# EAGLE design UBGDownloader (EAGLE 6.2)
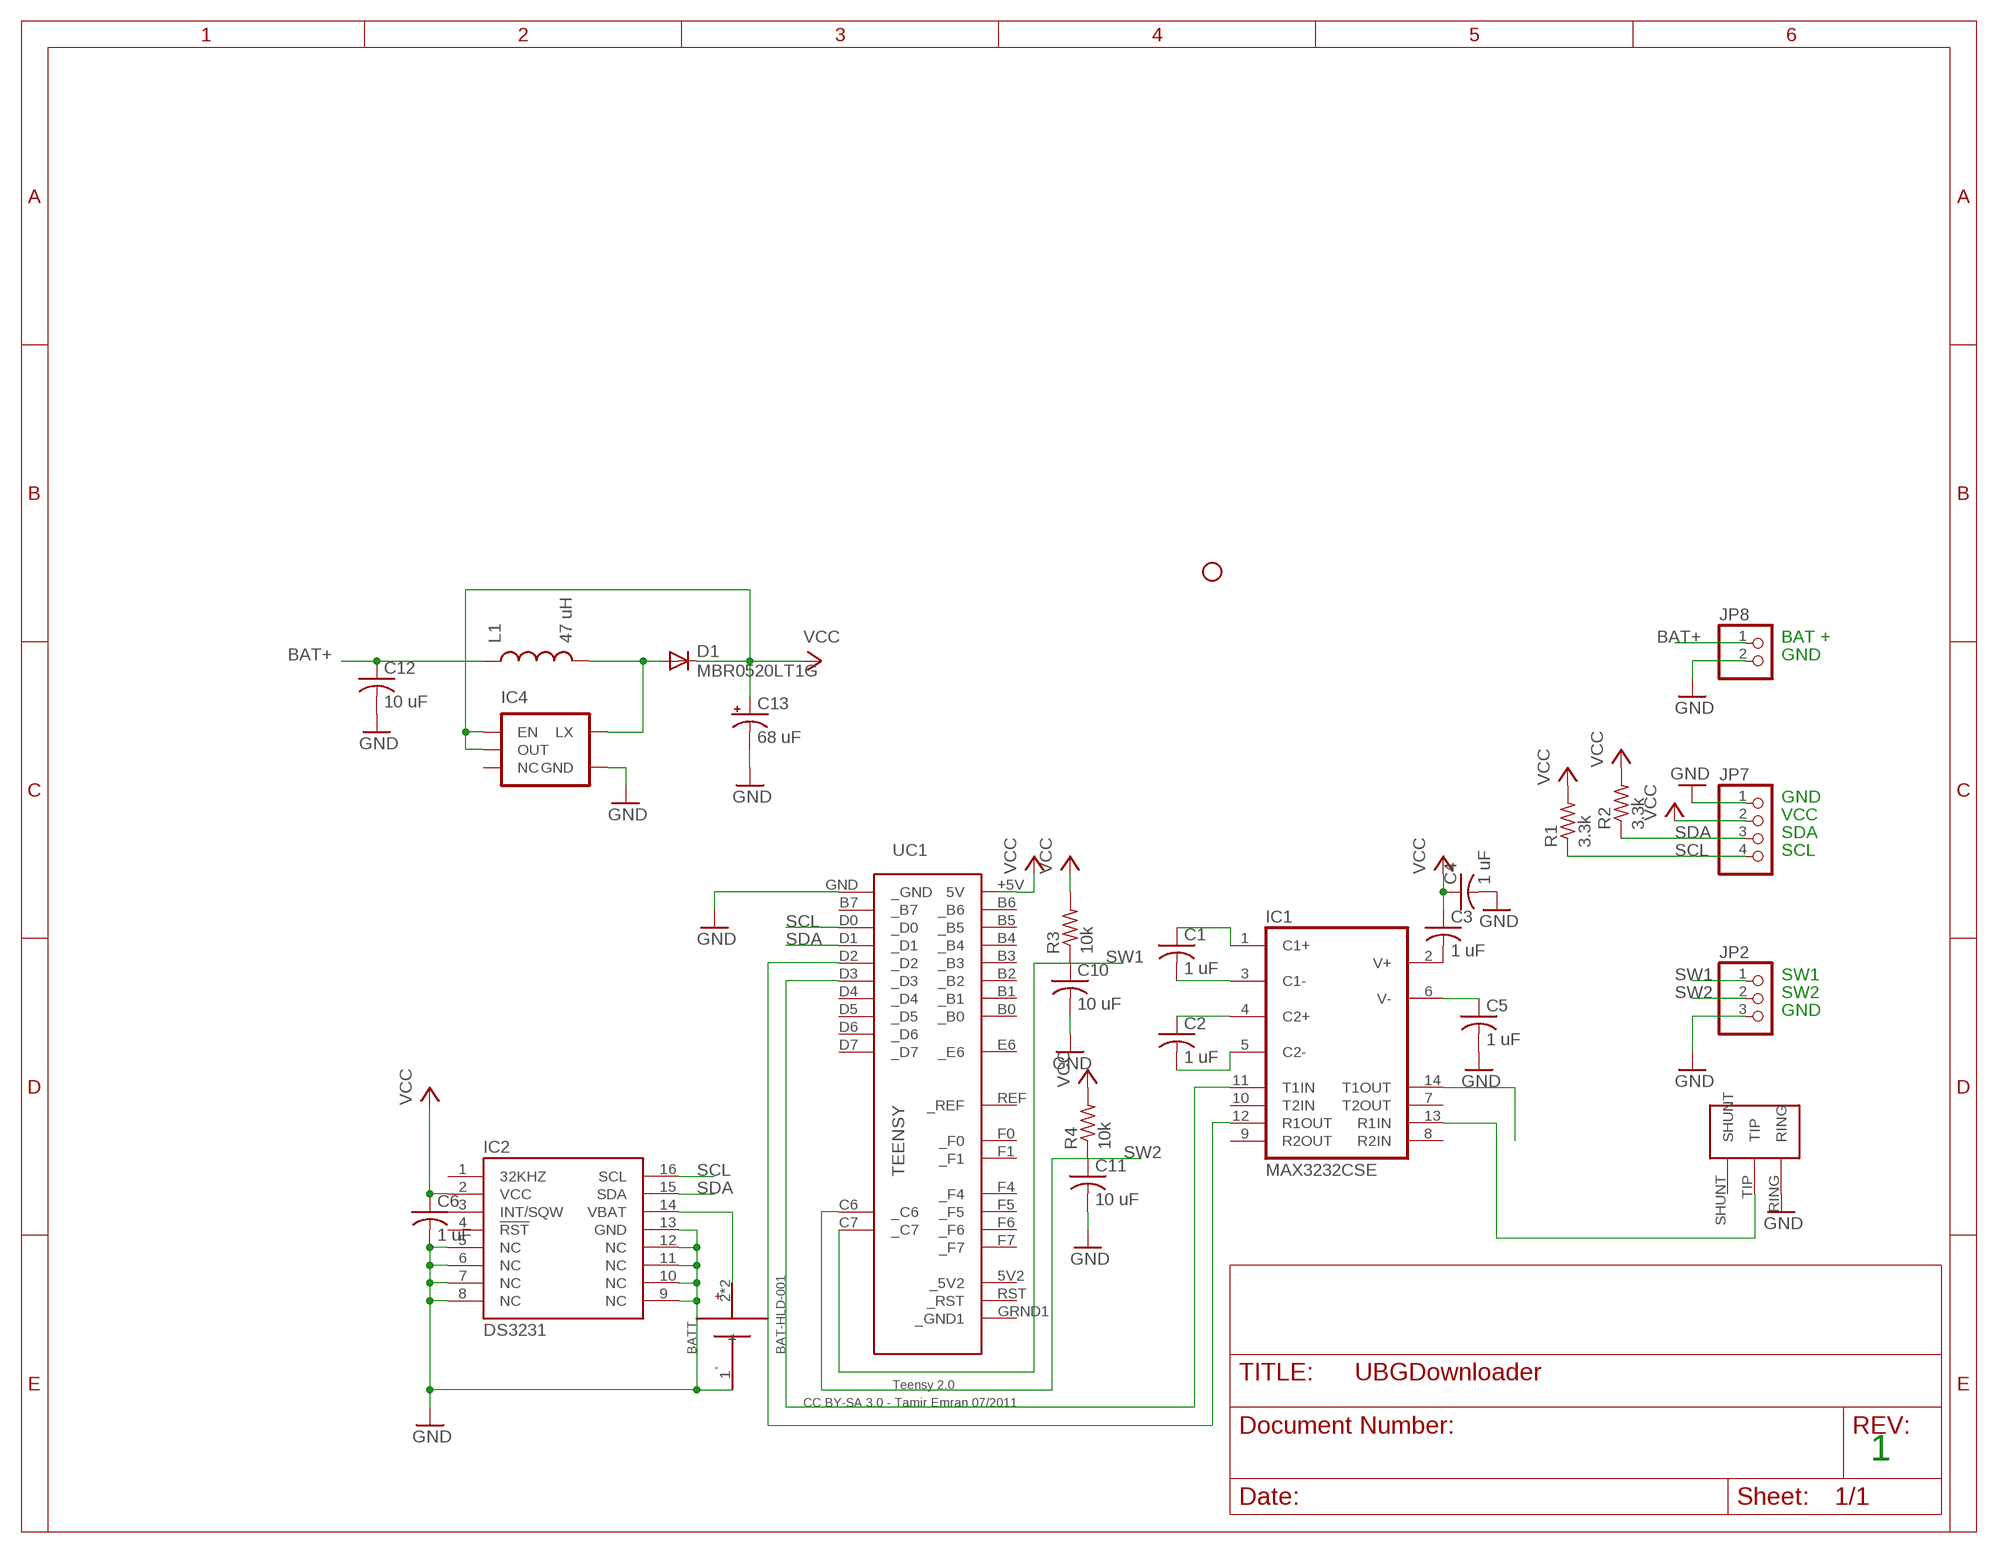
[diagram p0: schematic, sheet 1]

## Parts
BATT  BAT-HLD-001  [BAT-HLD-001]
C1  1 uF  C-USC0805K  [C0805K]
C2  1 uF  C-USC0805K  [C0805K]
C3  1 uF  C-USC0805K  [C0805K]
C4  1 uF  C-USC0805K  [C0805K]
C5  1 uF  C-USC0805K  [C0805K]
C6  1 uF  C-USC0805K  [C0805K]
C10  10 uF  C-USC0805K  [C0805K]
C11  10 uF  C-USC0805K  [C0805K]
C12  10 uF  C-USC0805K  [C0805K]
C13  68 uF  CPOL-USB/3528-21R  [B/3528-21R]
D1  MBR0520LT1G  CGRM4001-G  [SOD-123_MINI-SMA]
IC1  MAX3232CSE  [SO16]
IC2  DS3231  [SO-16]
IC4  V_REG_NCP1400SOT23-5  [SOT23-5]
JP2  PINHD-1X3  [1X03]
JP5  STAND-OFF  [STAND-OFF]
JP7  PINHD-1X4  [1X04]
JP8  PINHD-1X2  [1X02]
L1  47 uH  INDUCTORCDRH5D28R  [CDRH5D28R]
R1  3.3k  R-US_R0805  [R0805]
R2  3.3k  R-US_R0805  [R0805]
R3  10k  R-US_R0805  [R0805]
R4  10k  R-US_R0805  [R0805]
U$3  35RAPC2AVDEFAULT  [35RAPC2AV]
UC1  TEENSY  [TEENSY]

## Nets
BAT+: C12.1 JP8.1 L1.P$1
GND: BATT.1(-) C4.2 C5.2 C6.2 C10.2 C11.2 C12.2 C13.- IC2.5(NC) IC2.6(NC) IC2.7(NC) IC2.8(NC) IC2.9(NC) IC2.10(NC) IC2.11(NC) IC2.12(NC) IC2.13(GND) IC4.4(GND) JP2.3 JP7.1 JP8.2 U$3.RING UC1.GND(_GND)
N$3: BATT.2(+) BATT.3(+) IC2.14(VBAT)
N$4: C1.2 IC1.3(C1-)
N$5: C1.1 IC1.1(C1+)
N$6: C2.1 IC1.4(C2+)
N$7: C2.2 IC1.5(C2-)
N$8: C3.2 IC1.2(V+)
N$9: C5.1 IC1.6(V-)
N$10: IC1.13(R1IN) U$3.TIP
N$11: IC1.11(T1IN) UC1.D3(_D3)
N$12: IC1.12(R1OUT) UC1.D2(_D2)
N$16: IC1.14(T1OUT)
N$71: D1.A IC4.5(LX) L1.P$2
SCL: IC2.16(SCL) JP7.4 R1.1 UC1.D0(_D0)
SDA: IC2.15(SDA) JP7.3 R2.1 UC1.D1(_D1)
SW1: C10.1 JP2.1 R3.1 UC1.C7(_C7)
SW2: C11.1 JP2.2 R4.1 UC1.C6(_C6)
VCC: C3.1 C4.1 C6.1 C13.+ D1.C IC2.2(VCC) IC4.1(EN) IC4.2(OUT) JP7.2 R1.2 R2.2 R3.2 R4.2 UC1.+5V(5V)
Unconnected: IC1.7(T2OUT) IC1.8(R2IN) IC1.9(R2OUT) IC1.10(T2IN) IC2.1(32KHZ) IC2.3(INT/SQW) IC2.4(!RST) IC4.3(NC) U$3.SHUNT UC1.5V2(_5V2) UC1.B0(_B0) UC1.B1(_B1) UC1.B2(_B2) UC1.B3(_B3) UC1.B4(_B4) UC1.B5(_B5) UC1.B6(_B6) UC1.B7(_B7) UC1.D4(_D4) UC1.D5(_D5) UC1.D6(_D6) UC1.D7(_D7) UC1.E6(_E6) UC1.F0(_F0) UC1.F1(_F1) UC1.F4(_F4) UC1.F5(_F5) UC1.F6(_F6) UC1.F7(_F7) UC1.GRND1(_GND1) UC1.REF(_REF) UC1.RST(_RST)

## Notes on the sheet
- BAT +
- GND
- GND
- VCC
- SDA
- SCL
- SW1
- SW2
- GND
- 1

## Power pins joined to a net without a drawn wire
GND: IC1.15(GND)
VCC: IC1.16(VCC)

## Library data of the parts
BATT = Dan's Parts:BAT-HLD-001: LINX Technologies BAT-HLD-001
C1-C6 C10-C12 = resistor:C-US: CAPACITOR, American symbol
C13 = adafruit:CPOL-US: POLARIZED CAPACITOR, American symbol
D1 = diode:CGRM400*-G: Molded plasitc,JEDEC SOD-123/Mini SMA
IC1 = maxim:MAX3232*: True RS-232 Transceivers 3.0V to 5.5V, Low-Power up to 1Mbps, Using Four 0.1µF External Capacitors Source: http://pdfserv.maxim-ic.com/en/ds/MAX3222-MAX3241.pdf; MPN: MAX3232CSE; OC_FARNELL: 9725490; OC_NEWARK: 90C2890
IC2 = ds3231:DS3231: DS3231 RTC
IC4 = SparkFun-PowerIC:V_REG_NCP1400: Switching step-up voltage regulator NCP1400 switiching regulator takes single cell AA and outputs 100mA at 3.3V or 5V with minimal number of external components.
JP2 = adafruit:PINHD-1X3: PIN HEADER
JP5 = SparkFun-Electromechanical:STAND-OFF: #4 Stand Off
JP7 = pinhead:PINHD-1X4: PIN HEADER
JP8 = pinhead:PINHD-1X2: PIN HEADER
L1 = SparkFun-Passives:INDUCTOR: Inductors
R1-R4 = adafruit:R-US_: RESISTOR, American symbol
U$3 = dan:35RAPC2AV
UC1 = teensy:TEENSY: Teensy 2.0 Original Design by Clint Fisher Modified Design by Tamir Emran Licensed Under Creative Commons Attribution-ShareAlike 3.0 Unported (CC BY-SA 3.0)

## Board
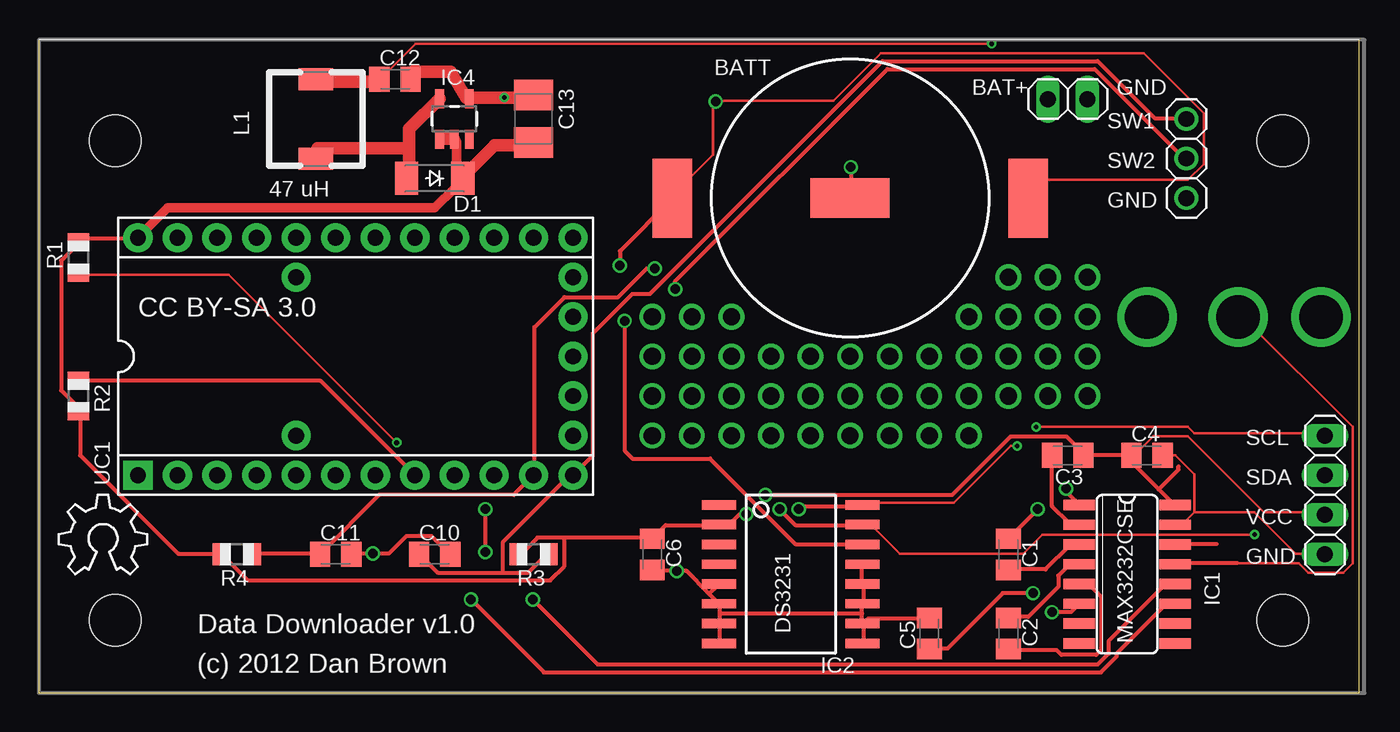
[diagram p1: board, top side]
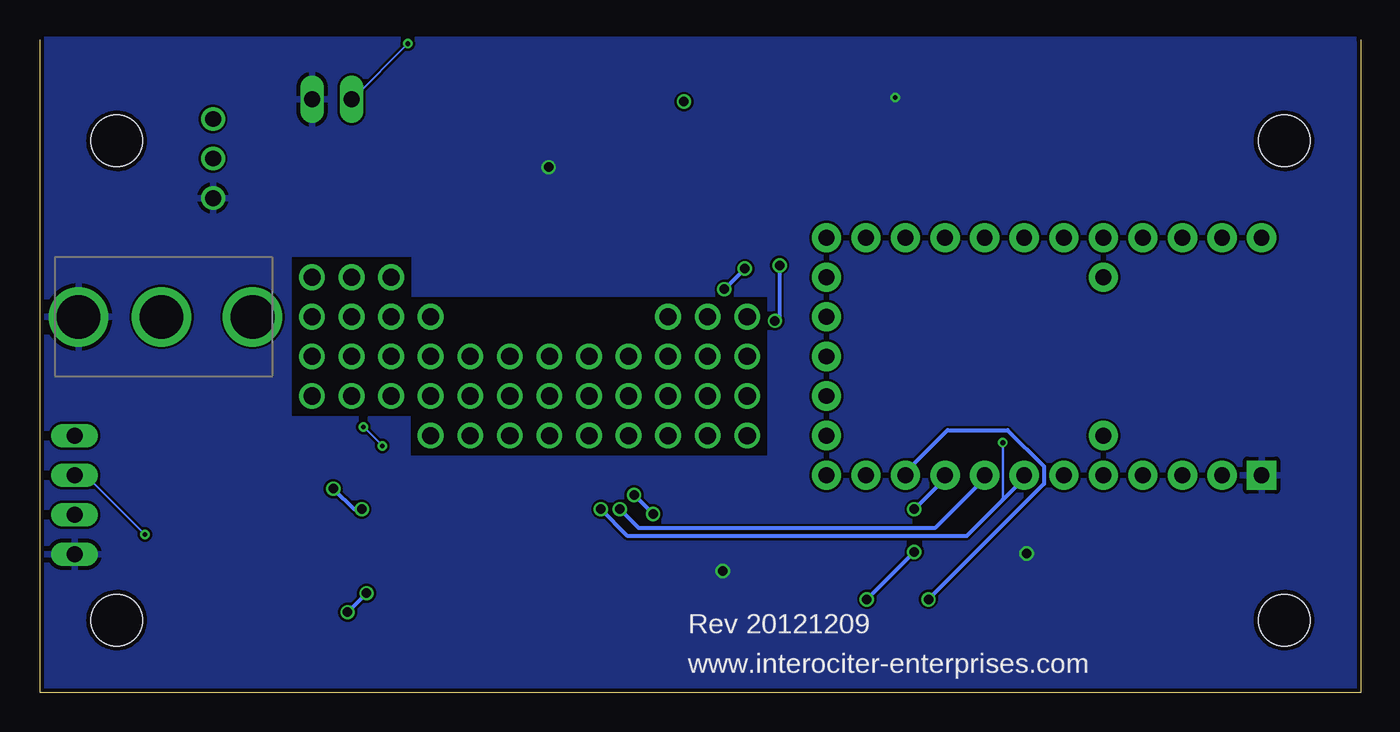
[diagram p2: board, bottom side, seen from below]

Size 84.76 x 41.9 mm. Coordinates in mm from the lower left corner, seen from the top.
Outline: 84.76,41.9 84.76,0 0,0 0,41.9
Copper layers (1*16): Top 0.035mm / dielectric 1.5mm / Bottom 0.035mm
Design rules: minimum track width 6mil, minimum drill 12mil, track to track 6mil, track to pad 6mil, pad to pad 6mil, via to via 6mil, smd to smd 0mil, copper to edge 10mil, drill to drill 10mil, minimum pad ring 10mil, minimum via ring 6mil, stop-mask expansion 2mil, vias tented up to drill 100mil, thermal gap 10mil
tRestrict: area 61,25.4 to 68.6,27.9; area 38.1,15.2 to 61,17.8
bRestrict: area 38.1,17.8 to 68.6,25.4; area 38.1,15.2 to 61,17.8; area 61,25.4 to 68.6,27.9

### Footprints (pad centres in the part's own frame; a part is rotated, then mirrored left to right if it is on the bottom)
BAT-HLD-001 = smd 5.08 x 2.54: 1 0,0 | smd 2.54 x 5.08: 2 -11.43,0; 3 11.43,0
C0805K = smd 1.3 x 1.6: 1 -1,0; 2 1,0
B/3528-21R = smd 1.95 x 2.5: + 1.525,0; - -1.525,0
SOD-123_MINI-SMA = smd 1.5 x 2.1: A 1.8,0; C -1.8,0
SO16 = smd 0.66 x 2.032: 1 -4.445,-3.073; 2 -3.175,-3.073; 3 -1.905,-3.073; 4 -0.635,-3.073; 5 0.635,-3.073; 6 1.905,-3.073; 7 3.175,-3.073; 8 4.445,-3.073; 9 4.445,3.073; 10 3.175,3.073; 11 1.905,3.073; 12 0.635,3.073; 13 -0.635,3.073; 14 -1.905,3.073; 15 -3.175,3.073; 16 -4.445,3.073
SO-16 = smd 0.6 x 2.2: 1 -4.445,-4.6; 2 -3.175,-4.6; 3 -1.905,-4.6; 4 -0.635,-4.6; 5 0.635,-4.6; 6 1.905,-4.6; 7 3.175,-4.6; 8 4.445,-4.6; 9 4.445,4.6; 10 3.175,4.6; 11 1.905,4.6; 12 0.635,4.6; 13 -0.635,4.6; 14 -1.905,4.6; 15 -3.175,4.6; 16 -4.445,4.6
SOT23-5 = smd 0.55 x 1.2: 1 -0.95,-1.3; 2 0,-1.3; 3 0.95,-1.3; 4 0.95,1.3; 5 -0.95,1.3
1X03 = drill 1.016: 1 -2.54,0; 2 0,0; 3 2.54,0
STAND-OFF = hole 3.302: 0,0
1X04 = drill 1.016 long: 1 -3.81,0; 2 -1.27,0; 3 1.27,0; 4 3.81,0
1X02 = drill 1.016 long: 1 -1.27,0; 2 1.27,0
CDRH5D28R = smd 2.2 x 1.4: P$1 0,2.55; P$2 0,-2.55
R0805 = smd 1.1 x 1.4: 1 -1,0; 2 1,0
35RAPC2AV = drill 2.8: RING 1.524,3.81; SHUNT 12.7,3.81; TIP 6.858,3.81
TEENSY = drill 1.016 pad 1.88: 5V2 13.97,-2.54; +5V -13.97,7.62; B0 -11.43,-7.62; B1 -8.89,-7.62; B2 -6.35,-7.62; B3 -3.81,-7.62; B4 8.89,7.62; B5 6.35,7.62; B6 3.81,7.62; B7 -1.27,-7.62; C6 11.43,-7.62; C7 13.97,-7.62; D0 1.27,-7.62; D1 3.81,-7.62; D2 6.35,-7.62; D3 8.89,-7.62; D4 13.97,5.08; D5 13.97,-5.08; D6 13.97,7.62; D7 11.43,7.62; E6 -3.81,-5.08; F0 -11.43,7.62; F1 -8.89,7.62; F4 -6.35,7.62; F5 -3.81,7.62; F6 -1.27,7.62; F7 1.27,7.62; GRND1 13.97,0; REF -3.81,5.08; RST 13.97,2.54 | drill 1.016 pad 1.88 square: GND -13.97,-7.62

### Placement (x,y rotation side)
BATT  52.07,31.75 180 top
C1  62.23,8.89 270 top
C2  62.23,3.81 270 top
C3  66.04,15.24 180 top
C4  71.12,15.24 0 top
C5  57.15,3.81 90 top
C6  39.37,8.89 270 top
C10  25.4,8.89 0 top
C11  19.05,8.89 0 top
C12  22.86,39.37 0 top
C13  31.75,36.83 270 top
D1  25.4,33.02 180 top
IC1  69.85,7.62 270 top
IC2  48.26,7.62 270 top
IC4  26.67,36.83 0 top
JP2  73.66,34.29 270 top
JP3  STAND-OFF  [STAND-OFF]  4.91,4.67 0 top
JP4  STAND-OFF  [STAND-OFF]  79.84,4.67 0 top
JP5  79.84,35.42 0 top
JP6  STAND-OFF  [STAND-OFF]  4.91,35.42 0 top
JP7  82.55,12.7 90 top
JP8  66.04,38.1 0 top
L1  17.78,36.83 0 top
R1  2.54,27.94 90 top
R2  2.54,19.05 270 top
R3  31.75,8.89 180 top
R4  12.7,8.89 180 top
U$2  [OSHW_6X200_NOTEXT]  1.27,7.62 0 top
U$3  83.82,20.32 0 bottom
UC1  20.32,21.59 0 top

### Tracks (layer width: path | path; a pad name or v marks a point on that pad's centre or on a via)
BAT+  (via drill 0.3)
  Top 0.152: 17.88,38.81 18.29,39.22 | 21.74,39.22 C12.1 21.95,39.42 24.18,41.66 v61.16,41.66
  Top 0.61: 18.29,39.22 17.78,39.22 L1.P$1
  Top 0.813: 18.29,39.22 21.74,39.22
  Bottom 0.152: v61.16,41.66 64.62,38.2 JP8.1
GND  (via drill 0.3, 0.61)
  Top 0.152: 27.64,38.2 IC4.4 27.43,38.2 | 31.7,38.2 C13.- | 23.98,39.85 C12.2 | C4.2 72.95,15.24 74.17,14.02 74.17,11.58 | 74.17,11.58 73.56,10.97 72.95,10.97 IC1.15 | 74.17,11.58 78.03,11.58 80.67,8.94 82.5,8.94 JP7.1
  Top 0.254: IC2.8 43.69,3.25 43.69,4.37 IC2.7 43.69,4.47 43.69,5.08 | 43.03,6.35 43.59,5.79 IC2.6 43.69,5.59 43.69,5.08 | 43.03,6.35 41.55,7.82 v40.95,7.82 39.42,7.82 C6.2 | 43.03,6.35 43.59,6.91 IC2.5 | IC2.13 52.83,8.23 52.83,7.11 IC2.12 52.93,6.91 52.93,5.79 IC2.11 52.83,5.59 52.83,5.08 | C5.2 57.1,4.78 53.24,4.78 52.93,4.47 IC2.10 | IC2.9 52.93,3.25 52.93,4.37 IC2.10 | 52.83,5.08 52.83,4.57 IC2.10 | 52.83,5.08 43.69,5.08 | C11.2 20.12,8.94 v21.44,8.94 22.45,8.94 23.57,10.06 25.2,10.06 26.31,8.94 C10.2 | v52.12,33.73 52.12,31.8 BATT.1
  Top 0.813: 31.7,38.2 v29.87,38.2 27.64,38.2 | 23.98,39.85 26.42,39.85 27.43,38.2
  pour Bottom: 0,41.91 85.09,41.91 85.09,0 0,0
N$1  (via drill 1.1)
  other vias: 52.07,19.05
N$2  (via drill 1.1)
  other vias: 54.61,19.05
N$3  (via drill 0.61)
  Top 0.152: BATT.3 40.64,31.9 43.28,34.54 43.28,37.8 v43.43,37.95 43.48,38 51,38 54.05,41.05 70.92,41.05 74.78,37.19 74.78,33.93 73.76,32.92 64.62,32.92 63.6,31.9 BATT.2
  Top 0.254: v37.59,23.88 37.59,15.54 38.1,15.04 43.08,15.04 48.56,9.55 52.83,9.55 IC2.14 | v37.29,27.43 37.29,28.35 40.64,31.7 BATT.3 | 63.5,31.7 BATT.2
  Bottom 0.254: v37.59,23.88 37.29,24.18 v37.29,27.43 37.39,27.43
N$4
  Top 0.254: C1.2 62.28,7.92 64.62,7.92 66.14,9.45 66.75,9.45 IC1.3
N$5  (via drill 0.61)
  Top 0.254: v64.11,11.79 62.28,9.96 C1.1 | v65.94,13.11 65.94,12.9 IC1.1
  Bottom 0.254: v64.11,11.79 64.62,11.79 v65.94,13.11
N$6
  Top 0.254: C2.1 62.28,4.88 63.5,4.88 65.43,6.81 65.43,7.52 66.14,8.23 66.75,8.23 IC1.4
N$7
  Top 0.254: C2.2 62.28,2.74 65.33,2.74 65.63,2.44 67.87,2.44 68.17,2.74 68.17,6.2 67.46,6.91 66.85,6.91 IC1.5
N$8
  Top 0.254: C3.2 65.02,15.24 65.02,11.99 66.14,10.87 66.75,10.87 IC1.2
N$9  (via drill 0.61)
  Top 0.254: v63.8,6.4 61.87,6.4 58.32,2.85 57.2,2.85 C5.1 | v65.02,5.18 66.24,5.18 IC1.6
  Bottom 0.254: v65.02,5.18 v63.8,6.4
N$10
  Top 0.152: 76.91,8.33 80.87,8.33 81.48,7.72 83.72,7.72 84.33,8.33 84.33,17.07 77.42,23.98 77.01,23.98 U$3.TIP
  Top 0.254: 76.91,8.33 72.95,8.33 IC1.13
N$11  (via drill 0.61)
  Top 0.254: v27.74,5.99 32.41,1.32 68.17,1.32 69.19,2.34 69.19,2.54 72.34,5.69 72.85,5.69 IC1.11
  Bottom 0.254: v27.74,5.99 20.32,13.41 20.32,14.53 22.66,16.87 26.52,16.87 29.16,14.22 29.16,14.02 UC1.D3
N$12  (via drill 0.61)
  Top 0.254: v31.7,5.99 35.87,1.83 67.97,1.83 68.68,2.54 68.68,3.35 72.24,6.91 72.85,6.91 IC1.12 | v28.65,11.79 v28.65,9.04
  Bottom 0.254: v28.65,9.04 v31.7,5.99 | v28.65,11.79 26.72,13.72 26.72,13.92 UC1.D2
N$14  (via drill 1.1)
  other vias: 49.53,19.05
N$16
  Top 0.254: 75.59,9.55 72.95,9.55 IC1.14
N$17  (via drill 1.1)
  other vias: 46.99,19.05
N$18  (via drill 1.1)
  other vias: 44.45,19.05
N$19  (via drill 1.1)
  other vias: 44.45,21.59
N$20  (via drill 1.1)
  other vias: 44.45,24.13
N$21  (via drill 1.1)
  other vias: 41.91,24.13
N$22  (via drill 1.1)
  other vias: 41.91,21.59
N$23  (via drill 1.1)
  other vias: 41.91,19.05
N$24  (via drill 1.1)
  other vias: 41.91,16.51
N$25  (via drill 1.1)
  other vias: 44.45,16.51
N$26  (via drill 1.1)
  other vias: 46.99,16.51
N$27  (via drill 1.1)
  other vias: 49.53,16.51
N$28  (via drill 1.1)
  other vias: 52.07,16.51
N$29  (via drill 1.1)
  other vias: 54.61,16.51
N$30  (via drill 1.1)
  other vias: 46.99,21.59
N$31  (via drill 1.1)
  other vias: 57.15,19.05
N$32  (via drill 1.1)
  other vias: 57.15,16.51
N$33  (via drill 1.1)
  other vias: 49.53,21.59
N$34  (via drill 1.1)
  other vias: 52.07,21.59
N$35  (via drill 1.1)
  other vias: 59.69,16.51
N$36  (via drill 1.1)
  other vias: 59.69,19.05
N$37  (via drill 1.1)
  other vias: 62.23,19.05
N$38  (via drill 1.1)
  other vias: 62.23,21.59
N$39  (via drill 1.1)
  other vias: 62.23,24.13
N$40  (via drill 1.1)
  other vias: 59.69,21.59
N$41  (via drill 1.1)
  other vias: 59.69,24.13
N$42  (via drill 1.1)
  other vias: 57.15,21.59
N$43  (via drill 1.1)
  other vias: 62.23,26.67
N$44  (via drill 1.1)
  other vias: 64.77,26.67
N$45  (via drill 1.1)
  other vias: 64.77,24.13
N$46  (via drill 1.1)
  other vias: 64.77,21.59
N$47  (via drill 1.1)
  other vias: 64.77,19.05
N$48  (via drill 1.1)
  other vias: 67.31,19.05
N$49  (via drill 1.1)
  other vias: 67.31,21.59
N$50  (via drill 1.1)
  other vias: 67.31,24.13
N$51  (via drill 1.1)
  other vias: 67.31,26.67
N$64  (via drill 1.1)
  other vias: 54.61,21.59
N$67  (via drill 1.1)
  other vias: 39.37,16.51
N$68  (via drill 1.1)
  other vias: 39.37,19.05
N$69  (via drill 1.1)
  other vias: 39.37,21.59
N$70  (via drill 1.1)
  other vias: 39.37,24.13
N$71
  Top 0.152: 25.6,38 IC4.5 | 23.77,33.12 D1.A
  Top 0.61: 17.88,34.95 17.78,34.95 L1.P$2
  Top 0.813: 23.77,33.12 23.77,34.95 | 17.88,34.95 23.77,34.95 | 23.77,34.95 23.77,36.18 IC4.5
SCL  (via drill 0.3, 0.61)
  Top 0.152: v22.96,16.05 12.19,26.82 2.64,26.82 R1.1 | v64.01,17.07 73.76,17.07 74.17,16.66 82.5,16.66 JP7.4 | v62.79,15.85 62.38,15.85 58.73,12.19 53.03,12.19 IC2.16
  Top 0.254: v48.77,11.79 48.97,11.99 52.83,11.99 IC2.16
  Bottom 0.152: 22.96,12.39 v22.96,16.05 | v62.79,15.85 v64.01,17.07
  Bottom 0.254: v48.77,11.79 47.04,10.06 25.3,10.06 22.96,12.39 21.64,13.72 21.64,13.92 UC1.D0
SDA  (via drill 0.3, 0.61)
  Top 0.152: v78.03,10.16 64.41,10.16 63.2,8.94 55.27,8.94 53.44,10.77 53.03,10.77 IC2.15
  Top 0.254: UC1.D1 18.09,20.02 2.54,20.02 R2.1 | v47.55,11.79 48.56,10.77 52.83,10.77 IC2.15
  Bottom 0.152: v78.03,10.16 81.69,13.82 82.5,13.82 JP7.3
  Bottom 0.254: v47.55,11.79 46.33,10.57 27.33,10.57 24.18,13.72 24.18,13.92 UC1.D1
SW1
  Top 0.254: 29.77,7.72 25.6,7.72 24.49,8.84 C10.1 | 29.77,7.72 31.39,7.72 32.51,8.84 32.72,8.84 R3.1 | JP2.1 73.66,36.88 71.63,36.88 67.97,40.54 54.15,40.54 39.22,25.6 38.1,25.6 35.56,23.06 35.56,15.24 UC1.C7 34.24,13.92 34.04,13.92 29.77,9.65 29.77,7.72
SW2  (via drill 0.61)
  Top 0.254: R4.1 13.72,8.94 17.98,8.94 C11.1 18.09,8.94 21.84,12.7 30.48,12.7 UC1.C6 31.8,14.02 31.8,23.47 33.73,25.4 37.19,25.4 39.01,27.23 v39.52,27.23 | v40.84,25.91 40.84,26.42 54.46,40.03 67.77,40.03 73.46,34.34 73.66,34.34 JP2.2
  Bottom 0.254: v39.52,27.23 v40.84,25.91
VCC  (via drill 0.61)
  Top 0.152: 6.5,29.26 UC1.+5V | JP7.2 82.5,11.58 78.64,11.58 73.76,16.46 71.53,16.46 70.31,15.24 C4.1 | 25.81,35.56 IC4.1 | 26.62,35.56 IC4.2 26.82,35.36 | 27.03,33.12 26.82,33.33 | 31.7,35.15 C13.+
  Top 0.254: 71.88,13.06 69.8,15.14 C4.1 C3.1 67.06,15.34 65.94,16.46 62.38,16.46 58.62,12.7 v46.63,12.7 | 71.88,13.06 72.85,12.09 IC1.16 | 73.15,14.53 73.15,14.33 71.88,13.06 | 33.73,9.96 39.32,9.96 C6.1 39.42,9.96 40.23,10.77 43.59,10.77 IC2.2 43.69,10.87 44.4,10.87 45.01,11.48 v45.41,11.48 | 33.73,9.96 32,9.96 30.99,8.94 30.79,8.94 R3.2 | UC1.+5V 6.3,29.16 2.85,29.16 2.64,28.96 R1.2 2.54,28.85 1.42,27.74 1.42,19.41 2.54,18.29 R2.2 2.64,17.98 2.64,15.24 8.94,8.94 11.68,8.94 R4.2 11.79,8.84 13.41,7.21 32.82,7.21 33.73,8.13 33.73,9.96
  Top 0.61: 6.5,29.26 6.5,29.36 8.26,31.11 25.4,31.11 26.67,32.38 27.2,32.38 D1.C 27.2,33.09 27.53,33.43 | 26.82,33.33 26.82,35.36 | 27.03,33.12 27.23,33.12
  Top 0.813: 26.62,35.56 25.81,35.56 | 31.7,35.15 29.26,35.15 27.53,33.43 27.23,33.12
  Bottom 0.254: v45.41,11.48 v46.63,12.7

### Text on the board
tPlace: BAT+ | GND | SW1 | SW2 | GND | SCL | SDA | VCC | GND | Data Downloader v1.0 | (c) 2012 Dan Brown
bPlace: Rev 20121209 | www.interociter-enterprises.com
